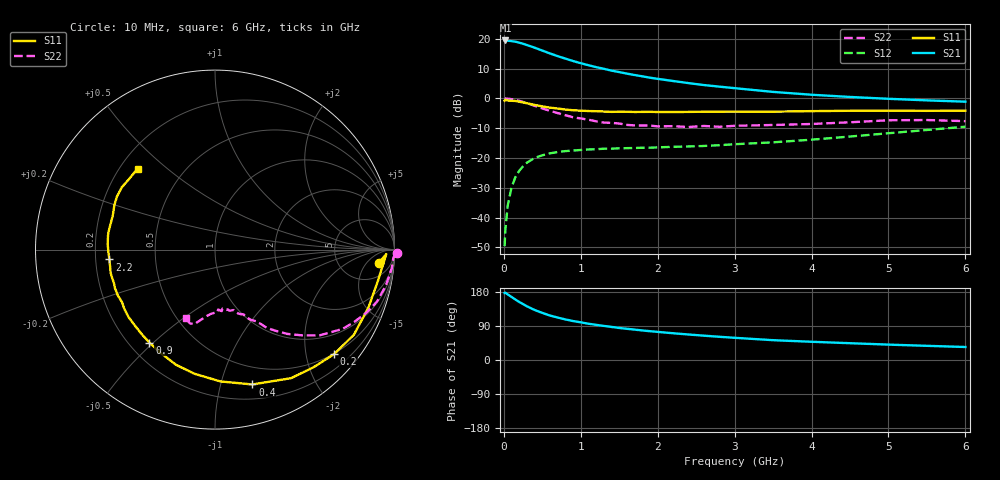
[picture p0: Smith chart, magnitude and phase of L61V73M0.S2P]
!  INFINEON TECHNOLOGIES Small Signal Semiconductors
! BFR380L3 , Si-NPN RF-Transistor in TSLP-3-1
!  Vce=1.75 V,  Ic=3 mA
! Common Emitter S-Parameters:  07. March 2005
#  GHz  S  MA  R  50
! f  S11  S21  S12  S22
! GHz  Mag  Ang  Mag  Ang  Mag  Ang  Mag  Ang
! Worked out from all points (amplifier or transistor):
!   36 points, 10 MHz to 6 GHz, reference 50 ohm
!   highest |S21| = 19.5 dB at 20 MHz (marker M1)
!   |S21| within 3 dB of that: start of sweep to 458.6 MHz
!   unconditionally stable (mu >= 1): 2.65 GHz to 4.728 GHz
!   at 250 MHz: K = 0.12, MSG = 20.6 dB, |S12| = -22.8 dB
!   at 1.4 GHz: K = 0.64, MSG = 13.1 dB, |S12| = -16.9 dB
!   at 6 GHz: K = 0.93, MSG = 4.2 dB, |S12| = -9.5 dB
!   S11 on the Smith chart (normalised r, x): 10 MHz: 12, -12; 200 MHz: 0.49, -2.58; 400 MHz: 0.33, -1.26; 900 MHz: 0.28, -0.49; 2.2 GHz: 0.26, -0.04; 6 GHz: 0.27, +0.40
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0.01  0.9172 -4.6  9.407 177.0  0.0033 87.1  1.014 -1.2
0.02  0.9545 -1.5  9.43 177.6  0.0063 88.6  0.9947 -2.5
0.05  0.9245 -10.8  9.363 173.1  0.0158 86.1  0.9903 -6.0
0.1  0.9137 -20.8  9.172 166.4  0.032 79.5  0.9728 -11.9
0.15  0.9076 -31.5  8.995 159.6  0.0476 73.1  0.9482 -17.8
0.2  0.8831 -41.2  8.662 153.1  0.0608 68.6  0.9145 -22.5
0.3  0.8323 -59.4  7.896 141.7  0.0835 59.4  0.8367 -31.9
0.4  0.7796 -74.5  7.126 132.0  0.1002 52.5  0.7522 -39.5
0.5  0.7353 -87.6  6.375 124.3  0.111 47.1  0.6802 -44.6
0.6  0.7011 -99.4  5.702 117.3  0.1196 43.0  0.6198 -49.3
0.7  0.6773 -108.8  5.142 112.0  0.1262 40.4  0.5679 -53.0
0.8  0.6512 -117.4  4.671 107.0  0.1305 37.8  0.5231 -56.5
0.9  0.6339 -125.2  4.254 102.8  0.1332 36.1  0.483 -58.6
1.1  0.6149 -136.7  3.618 95.7  0.139 34.4  0.4395 -63.0
1.5  0.5986 -154.7  2.774 84.6  0.1453 33.7  0.3792 -70.0
1.9  0.5958 -167.4  2.234 76.0  0.149 35.4  0.3504 -76.6
2.2  0.5912 -174.7  1.965 70.6  0.1541 37.8  0.3428 -78.8
2.8  0.601 172.9  1.58 61.3  0.164 43.7  0.3343 -87.0
3.5  0.6001 161.7  1.289 52.3  0.1833 49.8  0.3586 -93.6
4.5  0.621 151.7  1.06 44.3  0.2293 58.2  0.3981 -101.2
5.5  0.6194 140.4  0.929 37.4  0.2955 61.1  0.4342 -108.9
6  0.6242 133.7  0.883 34.3  0.3358 60.7  0.416 -113.1
